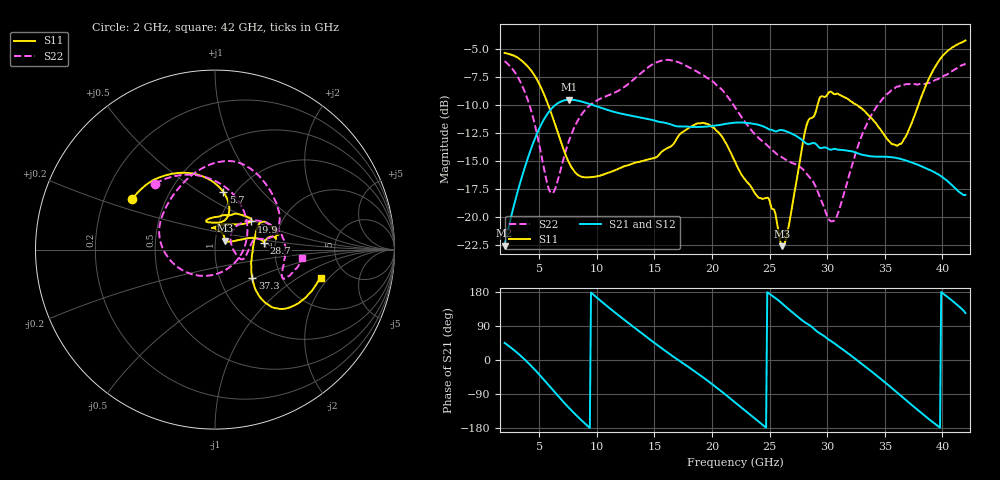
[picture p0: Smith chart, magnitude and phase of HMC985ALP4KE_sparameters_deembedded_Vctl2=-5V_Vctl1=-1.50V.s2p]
!s2p File: Measurements: S11, S21, S12, S22
# GHz S dB R 50.0
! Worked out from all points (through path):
!   401 points, 2 GHz to 42 GHz, reference 50 ohm
!   highest |S21| = -9.54 dB at 7.6 GHz (marker M1); lowest = -22.6 dB at 2 GHz (marker M2)
!   lowest |S11| = -22.6 dB at 26.1 GHz (marker M3), VSWR 1.16, Z = 55.6 + j5.47 ohm
!   |S11| at or under -10 dB: 5.791 GHz to 29.16 GHz (23.37 GHz wide, 134 % of centre); 32.58 GHz to 37.92 GHz (5.344 GHz wide, 15.2 % of centre)
!   |S22| runs from -20.4 to -6.0 dB; largest |S21 - S12| = 0.00032
!   S11 on the Smith chart (normalised r, x): 2 GHz: 0.32, +0.26; 5.7 GHz: 0.88, +0.63; 19.9 GHz: 1.41, +0.47; 28.7 GHz: 1.75, +0.15; 37.3 GHz: 1.43, -0.48; 42 GHz: 3.27, -1.66
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2  -5.35 148.4  -22.56 45.1  -22.57 45.1  -6.09 132.2
3.6  -6.15 121.9  -16.08 5.4  -16.09 5.4  -8.46 88.3
4.7  -7.54 100.9  -12.83 -28.1  -12.84 -28.1  -12.09 46.2
5.7  -9.76 81.9  -10.82 -62.2  -10.82 -62.2  -17.02 -18.4
6.3  -11.49 73.4  -10.09 -83.2  -10.10 -83.2  -17.70 -74.2
7.6  -15.17 71.2  -9.54 -126.8  -9.54 -126.8  -13.16 -150.2
8.7  -16.42 83.9  -9.70 -159.9  -9.70 -159.8  -10.82 -179.9
10.2  -16.33 99.3  -10.20 159.7  -10.21 159.7  -9.50 157.4
12.1  -15.60 107.3  -10.77 112.9  -10.78 112.9  -8.59 132.8
15.4  -14.46 81.2  -11.51 36.4  -11.51 36.4  -6.11 84.3
17.6  -12.32 53.5  -11.93 -10.7  -11.93 -10.6  -6.41 59.0
19.9  -11.89 38.0  -11.88 -61.1  -11.89 -61.1  -7.78 28.3
22  -15.06 52.5  -11.58 -111.9  -11.58 -111.9  -10.21 12.0
24.4  -18.39 98.2  -11.89 -171.2  -11.89 -171.2  -13.26 13.3
26.1  -22.60 41.3  -12.24 148.7  -12.25 148.7  -14.69 -2.7
28.7  -11.13 8.0  -13.41 86.6  -13.41 86.6  -16.70 -19.6
30.6  -9.03 14.5  -13.92 44.6  -13.93 44.6  -20.33 22.0
33.2  -10.51 30.7  -14.48 -14.8  -14.48 -14.8  -12.26 41.0
35.4  -13.25 8.2  -14.64 -68.6  -14.65 -68.5  -8.87 18.7
37.3  -11.71 -37.0  -15.12 -117.5  -15.12 -117.5  -8.14 -2.2
39.7  -6.06 -41.7  -16.23 -176.2  -16.23 -176.2  -7.64 -23.2
42  -4.24 -14.9  -18.03 123.9  -18.04 124.0  -6.29 -5.7
